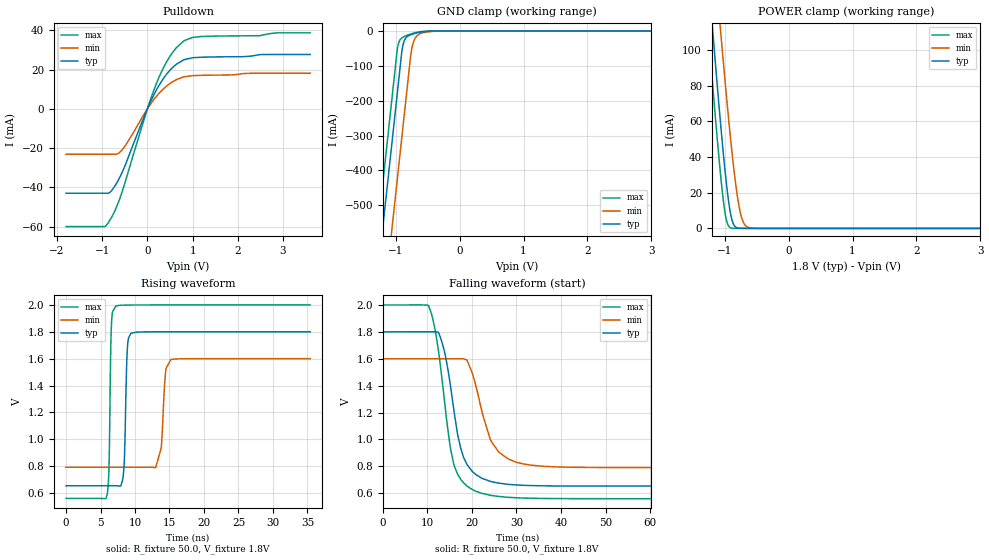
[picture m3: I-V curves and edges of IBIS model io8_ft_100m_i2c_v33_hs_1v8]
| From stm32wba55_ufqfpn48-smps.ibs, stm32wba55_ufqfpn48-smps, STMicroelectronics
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[Model]   io8_ft_100m_i2c_v33_hs_1v8
Model_type I/O_open_drain
Polarity   Non-Inverting
Enable   Active-Low
| CAP_THRESHOLD on pad IOFT is "UDTCAPC" :
| Rising=30.0% of vddiom   Falling=70.0% of vddiom
| C_comp min and max val. don't necessarily correlate with the min and max pvt
| but are the smallest and greatest pad capacitance found.
| var   typ   min   max
C_comp   2.22395pF  2.11500pF  2.41696pF
|C_comp_pulldown   2.22395pF  2.11500pF  2.41696pF
Vinl = 800.0mV
Vinh = 1.0V
Vmeas = 900.0mV   | Reference voltage for timing measurements
Cref  = 50.0pF   | Timing specification test load capacitance value
Rref  = 1.0MOhm   | Timing specification test load resistance value
Vref  = 990.0mV   | Timing specification test load voltage
[Model Spec]
| TIME_THRESHOLD on pin ZII2CV11 is "CMOS" :
| Rising=50.0% of vdd   Falling=50.0% of vdd
Vinl 697.50000mV 636.50000mV 765.50000mV
Vinh 1.08850V 942.50000mV 1.21750V
| variable   typ   min   max
[Temperature Range] 25.0 140.0 -40.0
| variable   typ   min   max
[Voltage Range] 1.8V 1.6V 2.0V
| variable   typ   min   max
[POWER Clamp Reference] 1.8V 1.6V 2.0V
| variable   typ   min   max
[GND Clamp Reference] 0V 0V 0V
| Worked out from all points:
|   slope of the pulldown table from 0 to 0.27 V, typ, clamps not added: 21.7 ohm
|   GND clamp passes 1 mA (typ) near -0.51 V on its own axis
|   POWER clamp passes 1 mA (typ) near -0.83 V on its own axis
|   rising waveform, R_fixture 50.0, V_fixture 1.8V: 20-80 % time 319ps typ, 504ps min, 243ps max; typ from 0.654 V to 1.8 V
|   falling waveform, R_fixture 50.0, V_fixture 1.8V: 20-80 % time 3.63ns typ, 4.45ns min, 3.48ns max; typ from 1.8 V to 0.654 V
[POWER Clamp]
-1.8V     396.4mA    438.1mA    365.5mA
-1.26V    143.5mA    194.6mA    112.6mA
-1.19V    112.3mA    164.2mA    81.56mA
-1.06V    57.23mA    109.3mA    28.68mA
-1.02V    41.75mA    93.06mA    15.5mA
-980mV    27.6mA     77.28mA    5.935mA
-910mV    8.693mA    51.24mA    382.3uA
-850mV    1.642mA    31.41mA    23.97uA
-760mV    69.41uA    9.714mA    358.6nA
-700mV    7.83uA     2.919mA    21.79nA
-620mV    424.6nA    410.3uA    573.9pA
3.6V      0A         0A         0A
[GND Clamp]
-1.8V     -1.583A    -1.83A     -1.456A
-1.43V    -953.9mA   -1.201A    -826.8mA
-1.24V    -630.9mA   -877.8mA   -503.8mA
-1.05V    -307.9mA   -554.8mA   -180.8mA
-970mV    -171.9mA   -418.8mA   -48.31mA
-910mV    -69.87mA   -316.8mA   -20.91mA
-880mV    -36.5mA    -265.8mA   -17.19mA
-830mV    -17.68mA   -180.8mA   -12.97mA
-750mV    -9.66mA    -53.66mA   -7.697mA
-690mV    -6.479mA   -19.19mA   -4.622mA
-600mV    -3.058mA   -6.478mA   -1.59mA
3.6V      1.281nA    1.39uA     517.2pA
| variable   typ   min   max
[Pullup Reference] 1.8V 1.6V 2.0V
| variable   typ   min   max
[Pulldown Reference] 0V 0V 0V
[Pulldown]
-1.8V     -42.97mA   -23.15mA   -59.99mA
-950mV    -42.97mA   -23.15mA   -59.99mA
-850mV    -42.87mA   -23.15mA   -57.45mA
-670mV    -37.41mA   -23.03mA   -49.3mA
-550mV    -31.91mA   -20.61mA   -41.6mA
10mV      539.8uA    356.7uA    722uA
230mV     10.88mA    7.174mA    14.64mA
500mV     19.69mA    12.93mA    26.79mA
790mV     24.78mA    16.15mA    34.26mA
1V        26.02mA    16.89mA    36.38mA
1.18V     26.27mA    17.05mA    36.82mA
3.6V      27.68mA    18.11mA    38.71mA
[Ramp]
dV/dt_r 687.66858mV/316.94147ps 484.89393mV/500.62649ps 863.98533mV/242.17354ps
dV/dt_f 687.69292mV/3.59946ns 484.93932mV/4.34796ns 864.00284mV/3.42605ns
R_load = 50.0
| Removed startup time: 0s 0s 0s  .
| Removed end time: 35.4ns.
[Rising Waveform]
R_fixture   = 50.0
V_fixture   = 1.8V
V_fixture_min = 1.6V
V_fixture_max = 2.0V
0s        653.8mV    791.8mV    560mV
5.95ns    653.8mV    791.8mV    585.3mV
6.6ns     653.8mV    791.8mV    1.871V
7.25ns    653.8mV    791.8mV    1.993V
8.35ns    760.3mV    791.8mV    1.998V
8.85ns    1.635V     791.8mV    1.999V
9.4ns     1.789V     791.8mV    1.999V
13ns      1.8V       789.7mV    2V
15.2ns    1.8V       1.594V     2V
35.4ns    1.8V       1.6V       2V
| Removed startup time: 0s 0s 0s  .
| Removed end time: 98.4ns.
[Falling Waveform]
R_fixture   = 50.0
V_fixture   = 1.8V
V_fixture_min = 1.6V
V_fixture_max = 2.0V
0s        1.8V       1.6V       2V
10.25ns   1.8V       1.6V       1.994V
11.75ns   1.8V       1.6V       1.811V
13.2ns    1.732V     1.6V       1.473V
15.9ns    1.23V      1.6V       819.5mV
18.1ns    868.8mV    1.6V       678.8mV
20.9ns    738.8mV    1.399V     615.4mV
24.5ns    685.8mV    976.9mV    583mV
30.75ns   660.9mV    824.1mV    565.5mV
98.4ns    653.8mV    791.8mV    560mV
